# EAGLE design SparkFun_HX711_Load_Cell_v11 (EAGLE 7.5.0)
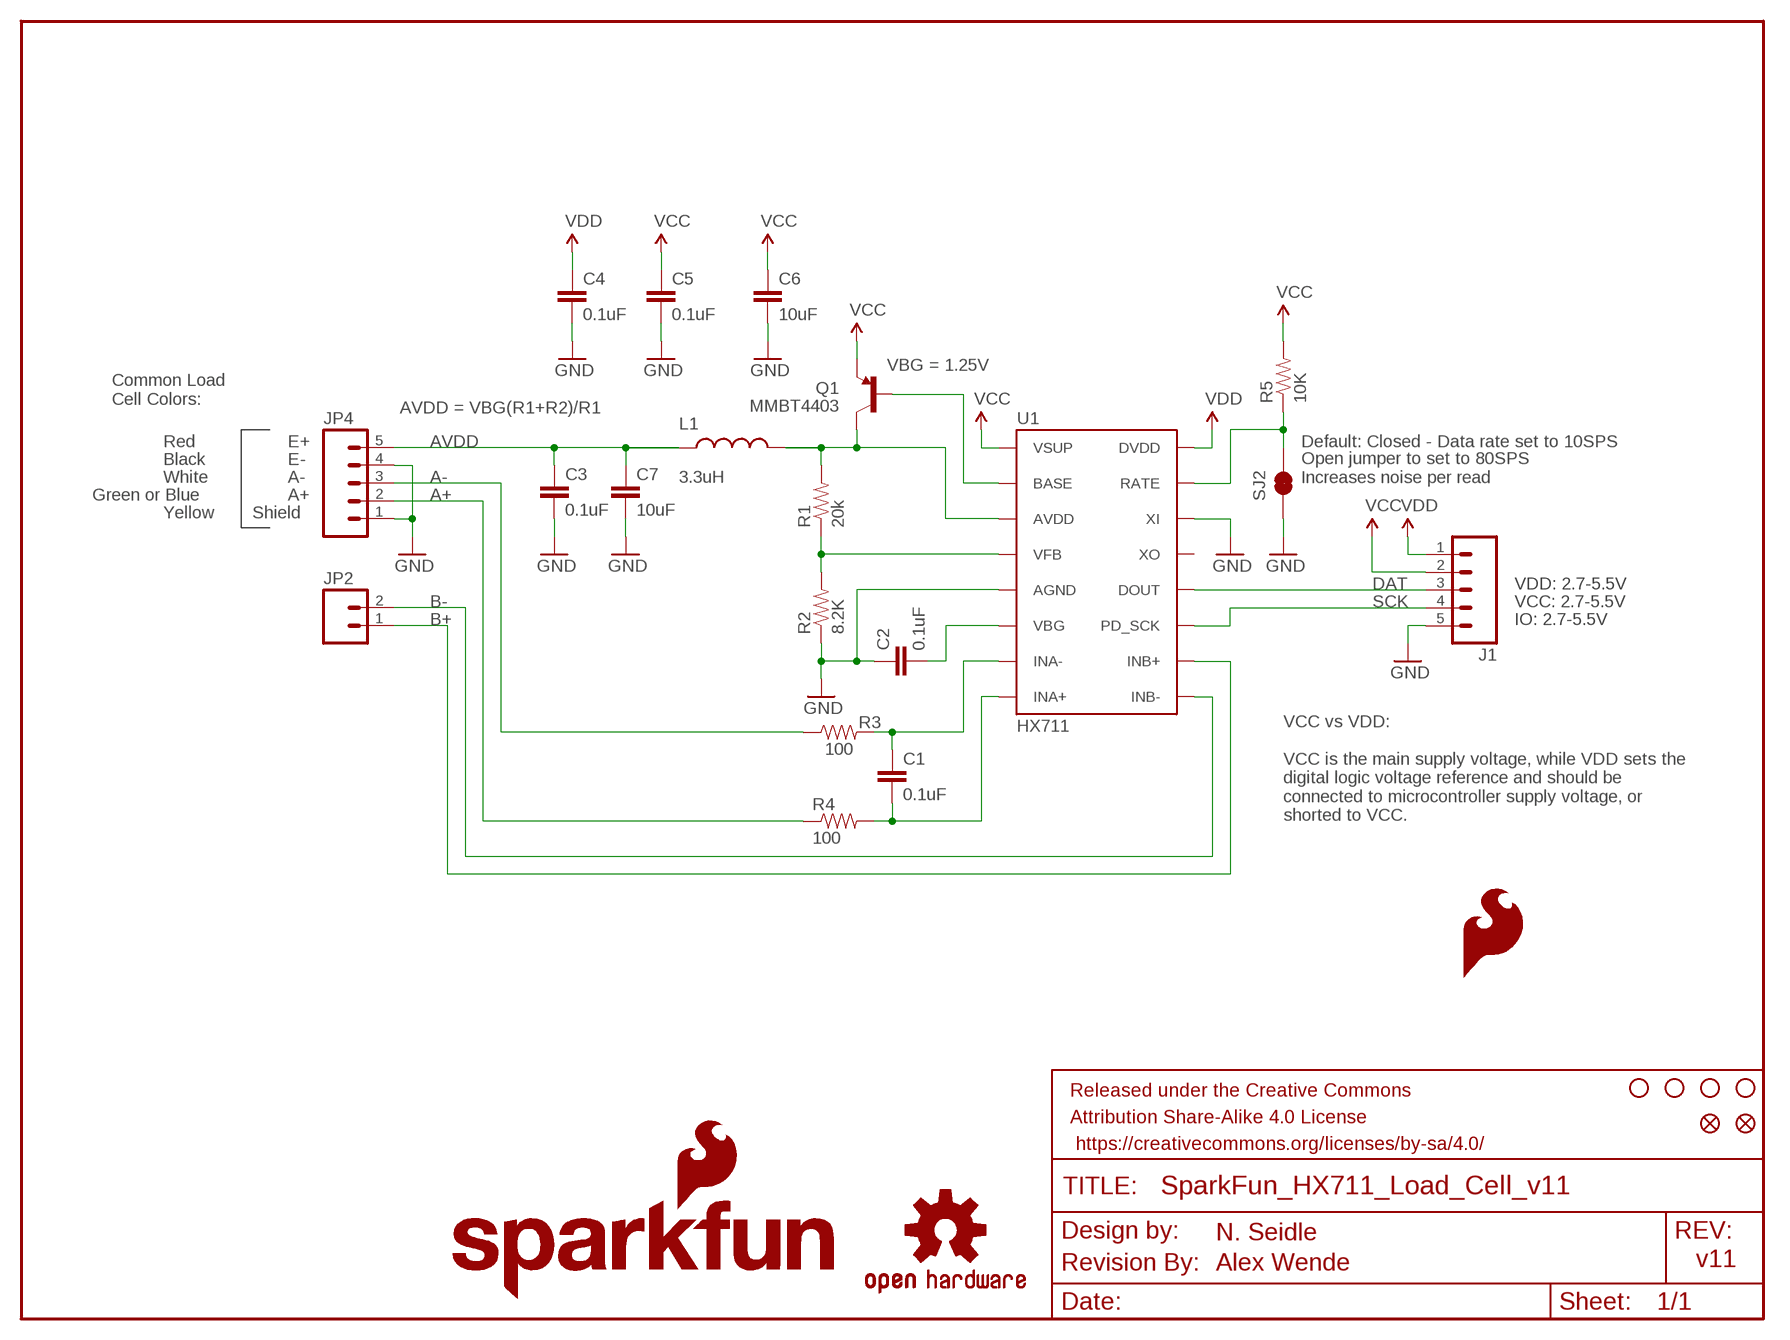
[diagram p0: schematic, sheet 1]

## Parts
C1  0.1uF  0.1UF-25V-5%(0603)  [0603-CAP]
C2  0.1uF  0.1UF-25V-5%(0603)  [0603-CAP]
C3  0.1uF  0.1UF-25V-5%(0603)  [0603-CAP]
C4  0.1uF  0.1UF-25V-5%(0603)  [0603-CAP]
C5  0.1uF  0.1UF-25V-5%(0603)  [0603-CAP]
C6  10uF  10UF50V20%(1210)  [1210]
C7  10uF  10UF50V20%(1210)  [1210]
FID1  FIDUCIAL1X2  [FIDUCIAL-1X2]
FID2  FIDUCIAL1X2  [FIDUCIAL-1X2]
FRAME1  FRAME-LETTER  [CREATIVE_COMMONS]
J1  M05PTH  [1X05]
JP2  M02PTH  [1X02]
JP4  M05PTH  [1X05]
L1  3.3uH  INDUCTOR0805-IND  [0805]
LOGO1  SFE_LOGO_NAME_FLAME.1_INCH  [SFE_LOGO_NAME_FLAME_.1]
LOGO3  SFE_LOGO_FLAME.1_INCH  [SFE_LOGO_FLAME_.1]
Q1  MMBT4403  TRANSISTOR_PNPMMBT4403  [SOT23-3]
R1  20k  20KOHM1/10W1%(0603)  [0603-RES]
R2  8.2K  8.2KOHM-1/10W-5%(0603)  [0603-RES]
R3  100  100OHM-1/10W-1%(0603)  [0603-RES]
R4  100  100OHM-1/10W-1%(0603)  [0603-RES]
R5  10K  10KOHM-1/10W-1%(0603)0603  [0603-RES]
SJ2  JUMPER-PAD-2-NC_BY_TRACE  [PAD-JUMPER-2-NC_BY_TRACE_YES_SILK]
STANDOFF1  STAND-OFF  [STAND-OFF]
STANDOFF2  STAND-OFF  [STAND-OFF]
STANDOFF3  STAND-OFF  [STAND-OFF]
STANDOFF4  STAND-OFF  [STAND-OFF]
U1  HX711  HX711HX711  [SO16]
U7  OSHW-LOGOS  [OSHW-LOGO-S]
U$1  REVISION  [REVISION]

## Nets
A+: JP4.2 R4.1
A-: JP4.3 R3.1
AVDD: C3.1 C7.1 JP4.5 L1.1
B+: JP2.1 U1.10(INB+)
B-: JP2.2 U1.9(INB-)
DAT: J1.3 U1.12(DOUT)
GND: C2.1 C3.2 C4.2 C5.2 C6.2 C7.2 J1.5 JP4.1 JP4.4 R2.1 SJ2.1 U1.5(AGND) U1.14(XI)
N$1: R5.1 SJ2.2 U1.15(RATE)
N$2: C1.1 R3.2 U1.7(INA-)
N$3: C1.2 R4.2 U1.8(INA+)
N$4: Q1.1(B) U1.2(BASE)
N$5: L1.2 Q1.3(C) R1.2 U1.3(AVDD)
N$6: R1.1 R2.2 U1.4(VFB)
N$7: C2.2 U1.6(VBG)
SCK: J1.4 U1.11(PD_SCK)
VCC: C5.1 C6.1 J1.2 Q1.2(E) R5.2 U1.1(VSUP)
VDD: C4.1 J1.1 U1.16(DVDD)
Unconnected: U1.13(XO)

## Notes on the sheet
- VBG = 1.25V
- Common Load
  Cell Colors:
- AVDD = VBG(R1+R2)/R1
- Red | E+ | Default: Closed - Data rate set to 10SPS
- Black | E-
- White | A-
- Open jumper to set to 80SPS
  Increases noise per read
- Green or Blue | A+
- Yellow | Shield
- VDD: 2.7-5.5V
- VCC: 2.7-5.5V
- IO: 2.7-5.5V
- VCC vs VDD:
  
  VCC is the main supply voltage, while VDD sets the
  digital logic voltage reference and should be
  connected to microcontroller supply voltage, or
  shorted to VCC.
- N. Seidle
- Alex Wende | v11

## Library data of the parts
C1-C5 = SparkFun-Capacitors:0.1UF-25V-5%(0603): CAP-08604; PROD_ID: CAP-08604
C6 C7 = SparkFun-Capacitors:10UF50V20%(1210): CAP-09824; PROD_ID: CAP-09824
FID1 FID2 = SparkFun-Aesthetics:FIDUCIAL: Fiducial Alignment Points
FRAME1 = SparkFun-Aesthetics:FRAME-LETTER: Schematic Frame
J1 JP4 = SparkFun-Connectors:M05: Header 5 Standard 5-pin 0.1" header. Use with straight break away headers (SKU : PRT-00116), right angle break away headers (PRT-00553), swiss pins (PRT-00743), machine pins (PRT-00117), and female headers (PRT-00115). Molex polarized connector foot print use with SKU : PRT-08230 with associated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
JP2 = SparkFun-Connectors:M02: Standard 2-pin 0.1" header. Use with
L1 = SparkFun-Passives:INDUCTOR: Inductors; PROD_ID: NDUC-13076
LOGO1 = SparkFun-Aesthetics:SFE_LOGO_NAME_FLAME: SFE Logo, name and flame
LOGO3 = SparkFun-Aesthetics:SFE_LOGO_FLAME: SFE Logo, flame only
Q1 = SparkFun-DiscreteSemi:TRANSISTOR_PNP: Generic PNP BJT Double check pinouts against datasheets- not all devices are the same! MMBT3906 - 40V 200mA SOT-23 (TRANS-08052) MMBT4403 - 40V 600mA SOT-23 (TRANS-09245); PROD_ID: TRANS-09245
R1 = SparkFun-Resistors:20KOHM1/10W1%(0603): RES-09383; PROD_ID: RES-09383
R2 = SparkFun-Resistors:8.2KOHM-1/10W-5%(0603): RES-10646; PROD_ID: RES-10646
R3 R4 = SparkFun-Resistors:100OHM-1/10W-1%(0603): RES-07863; PROD_ID: RES-07863
R5 = SparkFun-Resistors:10KOHM-1/10W-1%(0603): RES-00824; PROD_ID: RES-00824
SJ2 = SparkFun-Passives:JUMPER-PAD-2-NC_BY_TRACE
STANDOFF1-STANDOFF4 = SparkFun-Electromechanical:STAND-OFF: #4 Stand Off
U1 = Testing:HX711; PROD_ID: IC-12445
U7 = SparkFun-Aesthetics:OSHW-LOGO: Open Source Hardware Logo
U$1 = SparkFun-Aesthetics:REVISION

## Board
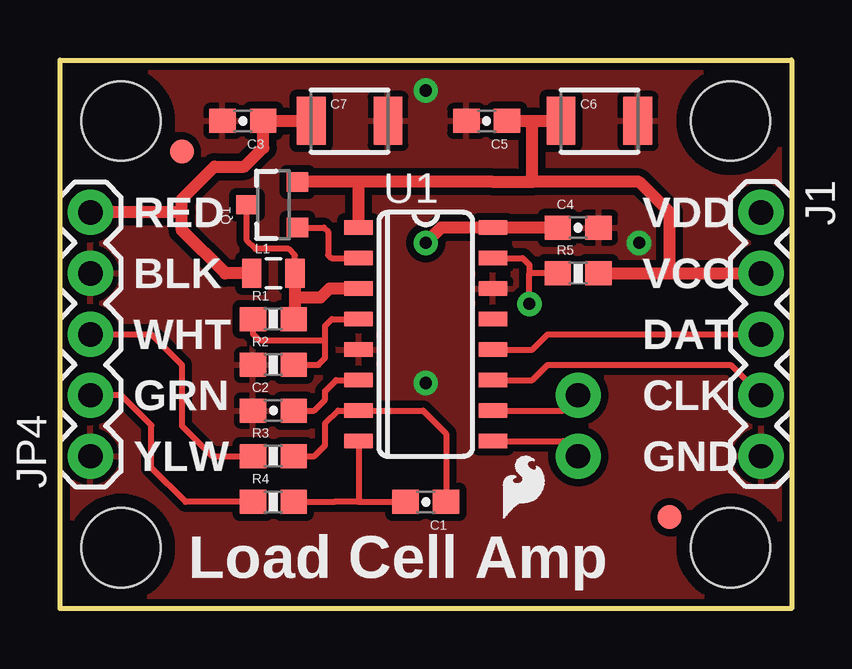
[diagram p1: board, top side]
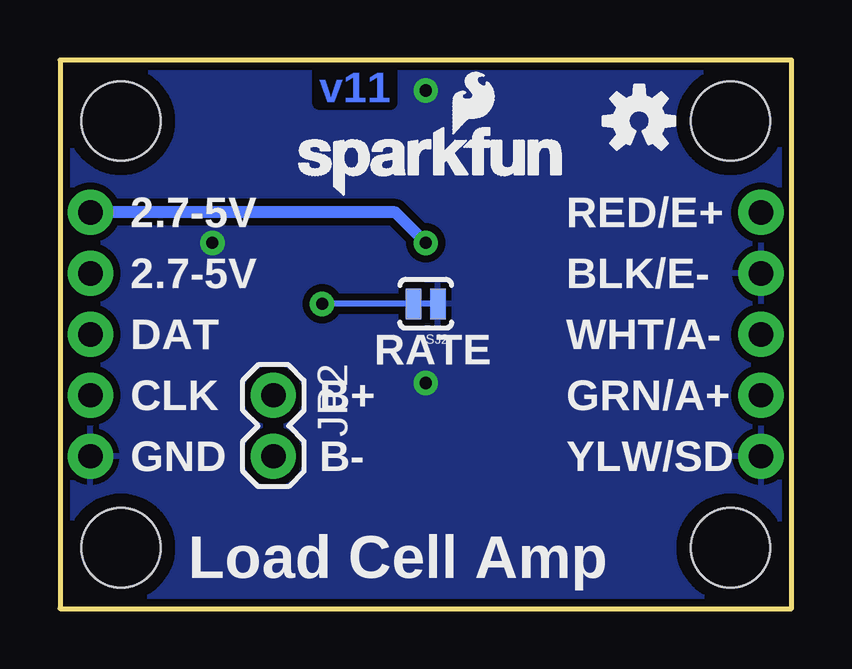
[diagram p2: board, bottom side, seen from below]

Size 30.48 x 22.86 mm. Coordinates in mm from the lower left corner, seen from the top.
Outline: 0,22.86 30.48,22.86 30.48,0 0,0 0,22.86
Copper layers (1*16): Top 0.035mm / dielectric 1.5mm / Bottom 0.035mm
Design rules "SparkFun-2-layer-STANDARD": minimum track width 10mil, minimum drill 20mil, track to track 10mil, track to pad 8mil, pad to pad 8mil, via to via 10mil, smd to smd 8mil, copper to edge 8mil, drill to drill 8mil, minimum pad ring 10mil, minimum via ring 10mil, stop-mask expansion 4mil, vias tented up to drill 25mil, thermal gap 10mil

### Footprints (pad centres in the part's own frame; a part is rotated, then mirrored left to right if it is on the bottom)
0603-CAP = smd 1.1 x 1: 1 -0.85,0; 2 0.85,0
1210 = smd 1.2 x 2: 1 -1.6,0; 2 1.6,0
FIDUCIAL-1X2 = smd 1 x 1: 1 0,0
1X05 = drill 1.016 pad 1.88: 1 0,0; 2 2.54,0; 3 5.08,0; 4 7.62,0; 5 10.16,0
1X02 = drill 1.016 pad 1.88: 1 0,0; 2 2.54,0
0805 = smd 0.8 x 1.2: 1 -0.9,0; 2 0.9,0
SOT23-3 = smd 0.8 x 0.9: 1 -0.95,-1; 2 0.95,-1; 3 0,1.1
0603-RES = smd 1.1 x 1: 1 -0.85,0; 2 0.85,0
PAD-JUMPER-2-NC_BY_TRACE_YES_SILK = smd 0.635 x 1.27: 1 -0.508,0; 2 0.508,0
STAND-OFF = hole 3.302: 0,0
SO16 = smd 0.6 x 1.2: 1 -4.445,-2.8; 2 -3.175,-2.8; 3 -1.905,-2.8; 4 -0.635,-2.8; 5 0.635,-2.8; 6 1.905,-2.8; 7 3.175,-2.8; 8 4.445,-2.8; 9 4.445,2.8; 10 3.175,2.8; 11 1.905,2.8; 12 0.635,2.8; 13 -0.635,2.8; 14 -1.905,2.8; 15 -3.175,2.8; 16 -4.445,2.8

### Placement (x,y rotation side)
C1  15.24,4.45 180 top
C2  8.89,8.26 0 top
C3  7.62,20.32 180 top
C4  21.59,15.88 0 top
C5  17.78,20.32 180 top
C6  22.48,20.32 0 top
C7  12.06,20.32 0 top
FID1  5.08,19.05 0 top
FID2  25.4,3.81 0 top
FRAME1  not placed on the board
J1  29.21,16.51 270 top
JP2  21.59,8.89 270 bottom
JP4  1.27,6.35 90 top
L1  8.89,13.97 0 top
LOGO1  20.95,17.14 0 bottom
LOGO3  18.16,3.43 0 top
Q1  8.89,16.83 90 top
R1  8.89,12.06 0 top
R2  8.89,10.16 0 top
R3  8.89,6.35 0 top
R4  8.89,4.45 0 top
R5  21.59,13.97 0 top
SJ2  15.24,12.7 180 bottom
STANDOFF1  2.54,2.54 0 top
STANDOFF2  27.94,2.54 0 top
STANDOFF3  2.54,20.32 0 top
STANDOFF4  27.94,20.32 0 top
U1  15.24,11.43 270 top
U7  6.35,20.32 0 bottom
U$1  not placed on the board

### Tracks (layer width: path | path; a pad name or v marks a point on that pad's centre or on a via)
A+
  Top 0.254: R4.1 5.23,4.45 3.81,5.87 3.81,7.63 2.55,8.89 JP4.2
A-
  Top 0.254: JP4.3 3.81,11.43 5.08,10.16 5.08,7.62 6.35,6.35 R3.1
AVDD
  Top 0.508: L1.1 6.88,13.97 5.08,15.77 5.08,16.51 | 5.08,16.51 JP4.5 | C7.1 C3.1 8.47,19.2 7.69,18.41 6.43,18.41 5.08,17.07 5.08,16.51
B+
  Top 0.254: U1.10 20.95,8.26 JP2.1
B-
  Top 0.254: U1.9 20.95,6.99 JP2.2
DAT
  Top 0.254: U1.12 19.68,10.79 20.32,11.43 J1.3
GND  (via drill 0.51)
  other vias: 15.24,9.4 24.13,15.24 15.24,21.59
  pour Top (isolate 0.305): 0,22.86 0,0 30.48,0 30.48,22.86
  pour Bottom (isolate 0.305): 0,22.86 0,0 30.48,0 30.48,22.86
N$1  (via drill 0.51)
  Top 0.254: U1.15 19.27,14.61 19.56,14.32 19.56,13.97 | R5.1 19.56,13.97 | v19.56,12.7 19.56,13.97
  Bottom 0.254: SJ2.2 v19.56,12.7
N$2
  Top 0.254: C1.1 16.09,7.29 15.13,8.26 U1.7 11.59,8.26 11.05,7.72 11.05,6.81 10.59,6.35 R3.2
N$3
  Top 0.254: R4.2 11.43,4.45 12.44,4.45 | 12.44,4.45 C1.2 | U1.8 12.44,4.45
N$4
  Top 0.254: Q1.1 10.99,15.88 11.18,15.7 11.18,14.73 11.3,14.61 U1.2
N$5
  Top 0.254: L1.2 9.79,14.72 9.53,14.99 8.15,14.99 7.79,15.35 Q1.3
  Top 0.508: L1.2 9.79,12.95 | 9.79,12.95 9.79,12.06 R1.2 | U1.3 11.23,13.34 10.85,12.95 9.79,12.95
N$6
  Top 0.254: R2.2 10.77,10.16 11.05,10.44 11.05,11.18 | 11.05,11.18 11.05,11.78 11.33,12.06 U1.4 | R1.1 8.04,11.45 8.31,11.18 11.05,11.18
N$7
  Top 0.254: C2.2 10.59,8.26 11.05,8.71 11.05,9.07 11.51,9.53 U1.6
SCK
  Top 0.254: U1.11 19.68,9.53 20.32,10.16 27.94,10.16 J1.4
VCC
  Top 0.508: 18.03,17.78 12.44,17.78 | 12.44,17.78 Q1.2 | 18.04,17.77 18.03,17.78 | 19.68,17.78 24.13,17.78 25.4,16.51 25.4,13.97 | 25.4,13.97 J1.2 | U1.1 12.44,17.78 | C5.1 19.68,20.32 | 19.68,20.32 C6.1 | R5.2 25.4,13.97 | 18.03,17.78 19.68,17.78 | 19.68,17.78 19.68,20.32
VDD  (via drill 0.51)
  Top 0.508: U1.16 C4.1 15.88,15.88 v15.24,15.24
  Bottom 0.508: v15.24,15.24 16.51,16.51 J1.1

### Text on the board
Bottom: v11
tPlace: RED | VDD | BLK | VCC | WHT | DAT | GRN | CLK | YLW | GND | Load Cell Amp
bPlace: RED/E+ | 2.7-5V | BLK/E- | 2.7-5V | WHT/A- | DAT | RATE | GRN/A+ | B+ | CLK | YLW/SD | B- | GND | Load Cell Amp
Measures: Units are in inches
tDocu: N. Seidle | Alex Wende

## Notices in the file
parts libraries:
SparkFun-Aesthetics: Licensing: CC v3.0 Share-Alike You are welcome to use this library for commercial purposes.
SparkFun-Aesthetics: Released under the Creative Commons Attribution Share-Alike 4.0 License
SparkFun-Aesthetics: https://creativecommons.org/licenses/by-sa/4.0
